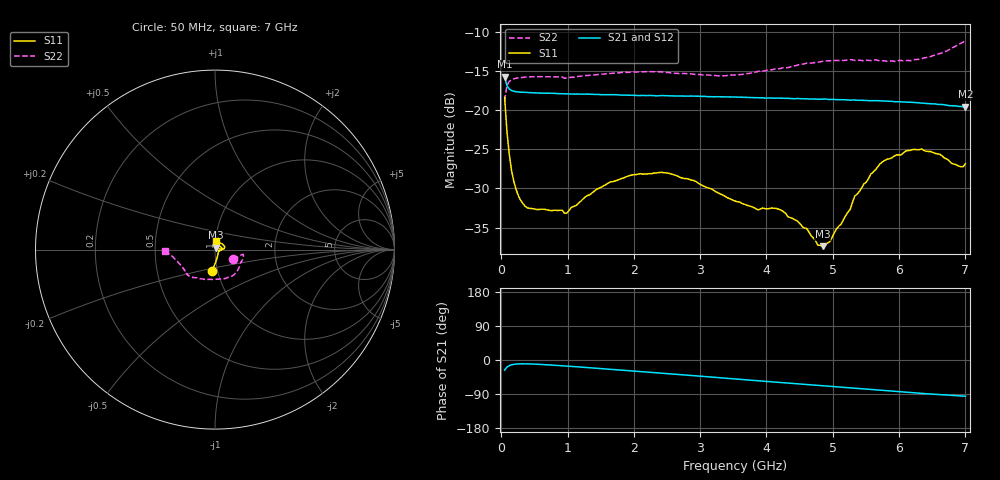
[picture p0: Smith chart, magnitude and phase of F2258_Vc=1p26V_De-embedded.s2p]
! Integrated Device Technology
! Corporate Headquarters
! 6024 Silver Creek Valley Road
! San Jose, CA 95138  USA
! Phone:  1-408-284-8200
! Toll Free:  1-800-223-1366
! Webpage:  http://www.idt.com/
! Timing and RF Division
! 515 Groton Road, Suite 102
! Westford, MA 01886-6024
! Device:  F2258
! Description: Voltage Variable RF Attenuator
! Frequency:  50.0 -  6000.00 MHz
! Package:  3x3 mm Thin QFN Plastic Package: 16 pin
! Ports:  2 RF, 2 DC
!  Pin  1  = NC
!  Pin  2  = NC
!  Pin  3  = RF2  = Port 2
!  Pin  4  = GND
!  Pin  5  = Vdd
!  Pin  6  = NC
!  Pin  7  = VCTRL
!  Pin  8  = NC
!  Pin  9  = GND
!  Pin 10  = RF1  = Port 1
!  Pin 11  = NC
!  Pin 12  = NC
!  Pin 13  = NC
!  Pin 14  = NC
!  Pin 15  = NC
!  Pin 16  = NC
! Vcntrl:  1.260 Volts
! Vdd:  +3.300 Volts
! Current:  1.166 mA
! Data:  The device was measured on a the F2258 evaluation board which has
!  individual transmission lines to the RF pins.  Data was collected
!  using a calibrated network analyzer.  The evaluation board was
!  de-embedded using a TRL calibration technique.
!  The reference plane is the edge of the package pin.
! Misc:  SN 10
!  Action Tracker AT0285
! Date Measured:  2014-12-10
! Date:  2016-01-13  MJV
! Note:
!  Integrated Device Technology supplies this data as a sample of measured
!  data at the package pin for this product.  Your particular data for this
!  product may vary.
!  Data was taken at 25 degrees C.
!  Integrated Device Technology reserves the right to change this data at anytime.
!Freq_(GHz)  S11M_(dB)  S11P_(deg)  S21M_(dB)  S21P_(deg)  S12M_(dB)  S12P_(deg)  S22M_(dB)  S22P_(deg)
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# GHz S dB R 50
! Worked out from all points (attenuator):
!   201 points, 50 MHz to 7 GHz, reference 50 ohm
!   highest |S21| = -15.76 dB at 50 MHz (marker M1); lowest = -19.6 dB at 7 GHz (marker M2)
!   lowest |S11| = -37.4 dB at 4.846 GHz (marker M3), VSWR 1.03, Z = 50.7 + j1.17 ohm
!   |S11| at or under -10 dB: start of sweep to end of sweep
!   |S22| runs from -18.8 to -11.1 dB; largest |S21 - S12| = 0.0013
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0.05  -18.36 -98.9  -15.76 -26.7  -15.81 -26.7  -18.80 -28.1
0.08475  -22.70 -87.7  -16.91 -18.9  -16.97 -18.9  -16.92 -13.8
0.15425  -27.70 -71.4  -17.52 -12.7  -17.56 -12.8  -16.16 -9.9
0.22375  -30.16 -59.1  -17.68 -10.7  -17.71 -10.7  -15.96 -9.6
0.328  -31.95 -43.1  -17.74 -10.0  -17.80 -10.0  -15.84 -11.3
0.98825  -33.16 -19.9  -17.95 -16.1  -17.88 -16.1  -15.93 -27.4
1.2315  -31.36 -12.2  -17.98 -19.1  -17.92 -19.1  -15.65 -33.1
1.6485  -29.17 -5.1  -18.06 -24.6  -18.00 -24.6  -15.34 -42.6
2.37825  -27.98 10.7  -18.19 -34.2  -18.12 -34.3  -15.13 -59.0
2.8995  -28.99 27.6  -18.24 -41.4  -18.20 -41.4  -15.44 -73.2
3.525  -31.61 60.7  -18.35 -50.0  -18.31 -50.1  -15.54 -96.5
3.8725  -32.76 84.9  -18.46 -54.8  -18.40 -54.9  -15.09 -109.7
4.22  -32.78 95.2  -18.50 -59.6  -18.47 -59.7  -14.70 -120.0
4.7065  -36.32 77.4  -18.60 -66.1  -18.57 -66.2  -14.00 -129.9
4.8455  -37.37 58.5  -18.62 -68.0  -18.60 -68.1  -13.80 -132.1
4.94975  -36.83 40.6  -18.67 -69.4  -18.63 -69.5  -13.75 -133.2
5.332  -30.98 7.7  -18.73 -74.6  -18.71 -74.6  -13.69 -137.5
5.57525  -28.16 4.1  -18.82 -77.7  -18.77 -77.8  -13.70 -141.3
5.85325  -26.23 6.2  -18.89 -81.5  -18.85 -81.6  -13.77 -145.9
6.33975  -24.97 17.4  -19.13 -88.2  -19.13 -88.2  -13.47 -157.9
6.9305  -27.24 72.7  -19.55 -94.9  -19.53 -94.9  -11.50 -176.2
7  -26.86 84.8  -19.60 -95.4  -19.59 -95.5  -11.14 -178.6
